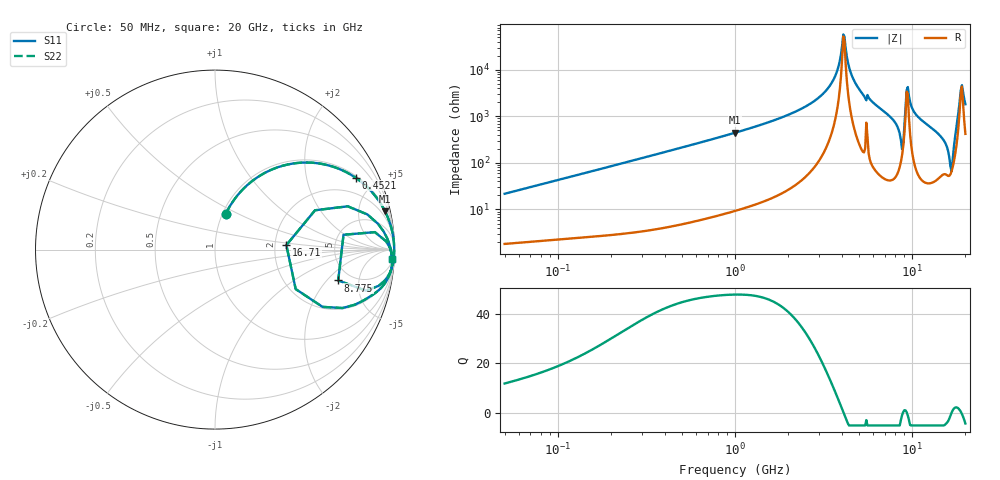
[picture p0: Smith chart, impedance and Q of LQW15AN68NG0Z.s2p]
!Murata Part Number: LQW15AN68NG0Z
!These Parameters are Measured in Series Mode Connection
!  o--[Z]--o
!Port1  Port2
!  o-------o
!Freq. Start=50[MHz] Stop=20[GHz], 401[Steps]
# Hz S RI R 50
!Freq.(Hz) S11(Real) S11(Imag) S21(Real) S21(Imag) S12(Real) S12(Imag) S22(Real) S22(Imag)
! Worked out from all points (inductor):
!   401 points, 50 MHz to 20 GHz, reference 50 ohm
!   read as one part in series: L = 68.6 nH near 51.52 MHz
!   highest Q = 47.7 at 1 GHz (marker M1), where L = 70.6 nH
!   self-resonance near 4.088 GHz
!   S11 on the Smith chart (normalised r, x): 50 MHz: 1.04, +0.43; 452.1 MHz: 1.09, +3.86; 8.775 GHz: 3.90, -2.69; 16.71 GHz: 2.31, +0.14; 20 GHz: 9, -35
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5e7  0.0604 0.1999  0.9396 -0.1999  0.9396 -0.1999  0.0604 0.1999
1.364002e8  0.262 0.4188  0.738 -0.4188  0.738 -0.4188  0.262 0.4188
3.721004e8  0.7104 0.4416  0.2896 -0.4416  0.2896 -0.4416  0.7104 0.4416
4.520922e8  0.7828 0.401  0.2172 -0.401  0.2172 -0.401  0.7828 0.401
1e9  0.9477 0.2125  0.0523 -0.2125  0.0523 -0.2125  0.9477 0.2125
2.728004e9  0.9957 0.05  0.00431 -0.05  0.00431 -0.05  0.9957 0.05
3.572216e9  0.9981 0.0171  0.00189 -0.0171  0.00189 -0.0171  0.9981 0.0171
4.087748e9  0.9984 0.000737  0.00158 -0.000737  0.00158 -0.000737  0.9984 0.000737
4.212059e9  0.9984 -0.00295  0.00159 0.00295  0.00159 0.00295  0.9984 -0.00295
4.539627e9  0.9982 -0.0124  0.00176 0.0124  0.00176 0.0124  0.9982 -0.0124
4.966507e9  0.9977 -0.0243  0.00229 0.0243  0.00229 0.0243  0.9977 -0.0243
7.442007e9  0.9865 -0.0965  0.0135 0.0965  0.0135 0.0965  0.9865 -0.0965
8.774992e9  0.6863 -0.1718  0.3137 0.1718  0.3137 0.1718  0.6863 -0.1718
9.316812e9  0.9747 0.00917  0.0253 -0.00917  0.0253 -0.00917  0.9747 0.00917
9.600142e9  0.9865 -0.0334  0.0135 0.0334  0.0135 0.0334  0.9865 -0.0334
1.050288e10  0.986 -0.0888  0.014 0.0888  0.014 0.0888  0.986 -0.0888
1.396067e10  0.9296 -0.209  0.0704 0.209  0.0704 0.209  0.9296 -0.209
1.573793e10  0.7771 -0.3076  0.2229 0.3076  0.2229 0.3076  0.7771 -0.3076
1.670968e10  0.3976 0.0249  0.6024 -0.0249  0.6024 -0.0249  0.3976 0.0249
1.747767e10  0.8493 0.1957  0.1507 -0.1957  0.1507 -0.1957  0.8493 0.1957
1.88369e10  0.9762 0.0124  0.0238 -0.0124  0.0238 -0.0124  0.9762 0.0124
2e10  0.9848 -0.0519  0.0152 0.0519  0.0152 0.0519  0.9848 -0.0519
